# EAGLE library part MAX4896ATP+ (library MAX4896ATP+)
Gate Drivers Space-Saving, 8-Channel Relay/Load Driver Source: Datasheet
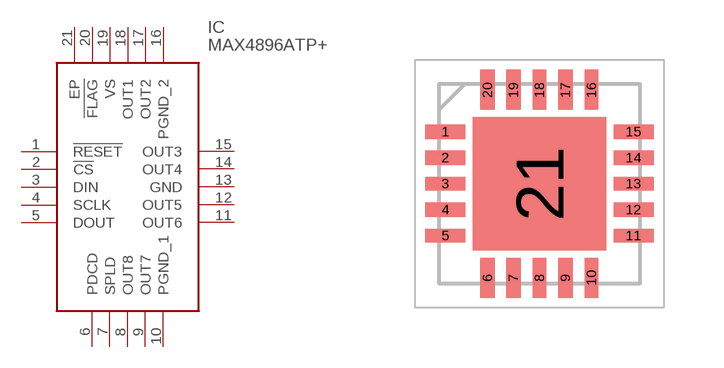
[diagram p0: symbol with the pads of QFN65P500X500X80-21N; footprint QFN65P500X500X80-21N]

Designator prefix IC

## MAX4896ATP+ (Arrow_Part_Number: MAX4896ATP+; Arrow_Price-Stock: https://www.arrow.com/en/products/max4896atp/maxim-integrated?region=nac; Description: Gate Drivers Space-Saving, 8-Channel Relay/Load Driver; Height: 0.8mm; Manufacturer_Name: Maxim Integrated; Manufacturer_Part_Number: MAX4896ATP+; Mouser_Part_Number: 700-MAX4896ATP; Mouser_Price-Stock: https://www.mouser.co.uk/ProductDetail/Maxim-Integrated/MAX4896ATP%2b?qs=1THa7WoU59EJbmvW8XRsRg%3D%3D)  [QFN65P500X500X80-21N]
1  !RESET
2  !CS
3  DIN
4  SCLK
5  DOUT
6  PDCD
7  SPLD
8  OUT8
9  OUT7
10  PGND_1
11  OUT6
12  OUT5
13  GND
14  OUT4
15  OUT3
16  PGND_2
17  OUT2
18  OUT1
19  VS
20  !FLAG
21  EP

## Footprint QFN65P500X500X80-21N (pad centres in mm)
T2055+5_1
smd 1 x 0.35: 1 -2.35,1.3; 2 -2.35,0.65; 3 -2.35,0; 4 -2.35,-0.65; 5 -2.35,-1.3; 11 2.35,-1.3; 12 2.35,-0.65; 13 2.35,0; 14 2.35,0.65; 15 2.35,1.3
smd 0.35 x 1: 6 -1.3,-2.35; 7 -0.65,-2.35; 8 0,-2.35; 9 0.65,-2.35; 10 1.3,-2.35; 16 1.3,2.35; 17 0.65,2.35; 18 0,2.35; 19 -0.65,2.35; 20 -1.3,2.35
smd 3.35 x 3.35: 21 0,0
